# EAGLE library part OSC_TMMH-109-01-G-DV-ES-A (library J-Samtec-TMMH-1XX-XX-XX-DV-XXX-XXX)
Samtec connector for SA.22c rubidium oscillator
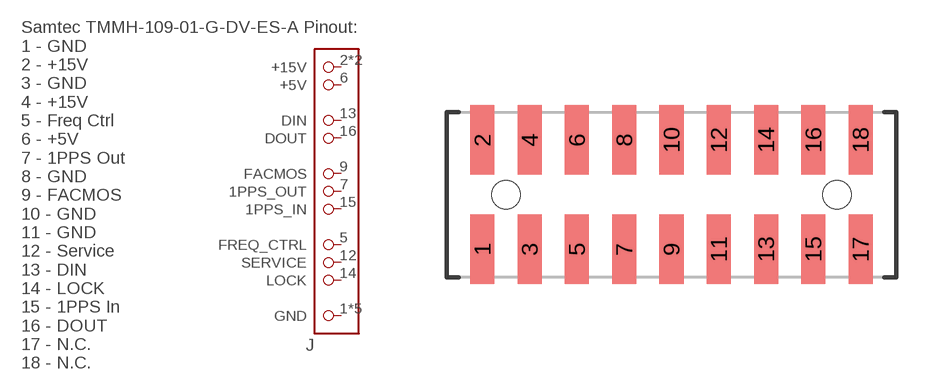
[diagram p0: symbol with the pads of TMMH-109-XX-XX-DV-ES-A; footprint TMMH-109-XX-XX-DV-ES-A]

Designator prefix J

## OSC_TMMH-109-01-G-DV-ES-A  [TMMH-109-XX-XX-DV-ES-A]
1  GND  pas
2  +15V  pas
3  GND  pas
4  +15V  pas
5  FREQ_CTRL  pas
6  +5V  pas
7  1PPS_OUT  pas
8  GND  pas
9  FACMOS  pas
10  GND  pas
11  GND  pas
12  SERVICE  pas
13  DIN  pas
14  LOCK  pas
15  1PPS_IN  pas
16  DOUT  pas

## Footprint TMMH-109-XX-XX-DV-ES-A (pad centres in mm)
2.00 mm SMT Header Source: Samtec TMMH-109-01-G-DV-ES-A
smd 1.016 x 2.94: 1 -8,-2.315; 2 -8,2.315; 3 -6,-2.315; 4 -6,2.315; 5 -4,-2.315; 6 -4,2.315; 7 -2,-2.315; 8 -2,2.315; 9 0,-2.315; 10 0,2.315; 11 2,-2.315; 12 2,2.315; 13 4,-2.315; 14 4,2.315; 15 6,-2.315; 16 6,2.315; 17 8,-2.315; 18 8,2.315
hole 1.19 at -7,0
hole 1.19 at 7,0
